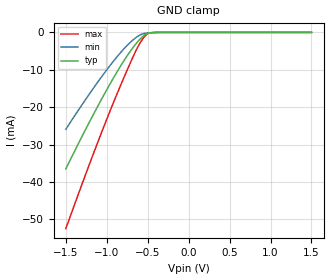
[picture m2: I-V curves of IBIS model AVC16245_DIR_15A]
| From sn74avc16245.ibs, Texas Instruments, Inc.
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[Model]   AVC16245_DIR_15A
Model_type  Input
Vinl = 0.49
Vinh = 1.04
| variable   typ   min   max
C_comp   1.87pF   1.50pF   2.11pF
[Temperature Range]   40   100   -40
| Ambient temperature   25   85   -40
[Voltage range]   1.5   1.4   1.6
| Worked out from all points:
|   GND clamp passes 1 mA (typ) near -0.56 V on its own axis
[GND Clamp]
| AVC16245_DIR_15A
|   Voltage   I(typ)   I(min)   I(max)
-1.5V     -36.47mA   -25.91mA   -52.48mA
-1.15V    -21.4mA    -14.52mA   -31.68mA
-1V       -15.33mA   -10.01mA   -23.22mA
-865mV    -10.22mA   -6.27mA    -15.95mA
-740mV    -5.914mA   -3.248mA   -9.541mA
-635mV    -2.815mA   -1.258mA   -4.517mA
-570mV    -1.285mA   -459.3uA   -2.031mA
-510mV    -341.5uA   -188.3uA   -518uA
-480mV    -166.9uA   -118.3uA   -185.6uA
-385mV    -13.73uA   -21.91uA   -7.311uA
1.5V      674.1pA    10.89nA    23.96pA
